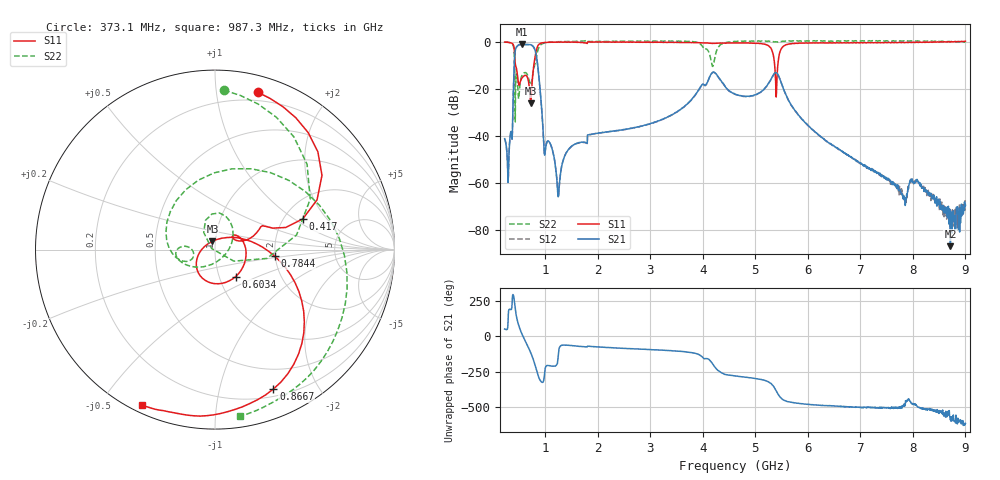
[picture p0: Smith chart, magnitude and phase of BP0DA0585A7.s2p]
!Agilent Technologies,E8358A,US41080443,A.07.50.56
!Agilent E8358A: A.07.50.56
!Date: Friday, November 10, 2017 15:52:36
!Correction: S11(Full 2 Port(1,2))
!S21(Full 2 Port(1,2))
!S12(Full 2 Port(1,2))
!S22(Full 2 Port(1,2))
!S2P File: Measurements: S11, S21, S12, S22:
# Hz S  dB  R 50
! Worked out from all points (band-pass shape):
!   1601 points, 225 MHz to 9 GHz, reference 50 ohm
!   highest |S21| = -1.21 dB at 559.5 MHz (marker M1); lowest = -86.9 dB at 8.715 GHz (marker M2)
!   |S21| within 3 dB of the highest: 425.6 MHz to 812.3 MHz (386.7 MHz wide, 62.5 % of centre)
!   lowest |S11| = -26.2 dB at 724.1 MHz (marker M3), VSWR 1.10, Z = 48.4 + j4.55 ohm
!   |S11| at or under -10 dB: 432.4 MHz to 781.6 MHz (349.3 MHz wide, 57.5 % of centre); 5.368 GHz to 5.428 GHz (59.98 MHz wide, 1.11 % of centre)
!   |S22| runs from -34.1 to 0.5 dB; largest |S21 - S12| = 0.0083
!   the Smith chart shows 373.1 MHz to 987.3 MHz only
!   S11 on the Smith chart (normalised r, x): 373.1 MHz: 0.13, +1.30; 417 MHz: 2.52, +1.18; 603.4 MHz: 1.20, -0.37; 784.4 MHz: 1.98, -0.16; 866.7 MHz: 0.27, -1.47; 987.3 MHz: 0.03, -0.64
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2.25e8  -0.22 138.0  -41.28 52.7  -41.32 52.7  -0.15 148.8
3.237188e8  -0.45 105.1  -41.87 -167.8  -41.98 -167.4  -0.43 119.9
3.730781e8  -0.83 74.8  -38.59 -86.4  -38.67 -86.2  -1.02 86.7
4.169531e8  -5.70 19.3  -6.28 -131.4  -6.36 -131.3  -10.67 -9.7
4.937344e8  -18.39 28.5  -1.42 78.2  -1.50 78.3  -24.34 -56.8
5.595469e8  -15.33 1.7  -1.21 13.9  -1.29 14.0  -14.20 -157.6
6.034219e8  -14.45 -52.5  -1.22 -21.0  -1.30 -21.0  -13.23 -170.1
7.240781e8  -26.21 106.6  -1.37 -115.8  -1.44 -115.7  -18.29 -166.4
7.844062e8  -9.53 -6.2  -2.57 -177.0  -2.63 -177.0  -11.27 169.7
8.666719e8  -1.49 -67.3  -12.43 79.1  -12.48 79.3  -3.16 5.3
9.873281e8  -0.40 -115.1  -48.28 107.0  -48.26 106.5  -0.55 -81.6
1.250578e9  -0.21 -154.1  -65.69 -118.1  -65.60 -122.0  -0.06 -120.7
1.689328e9  -0.37 166.8  -42.75 -70.5  -42.85 -70.4  0.20 -126.7
3.153656e9  -0.28 146.0  -33.70 -95.4  -33.73 -94.8  0.22 -152.8
4.140844e9  -0.71 117.1  -14.44 -171.3  -14.57 -171.0  -6.45 123.4
4.321828e9  -0.62 113.8  -15.88 112.0  -16.04 112.0  -1.64 -88.2
4.6125e9  -0.58 104.2  -22.34 81.6  -22.35 82.0  0.05 -124.3
5.396766e9  -23.57 -78.8  -13.16 -23.4  -13.21 -23.6  -0.11 -142.8
6.076828e9  -0.62 79.9  -37.26 -120.6  -37.32 -121.2  0.19 -152.7
7.541156e9  -0.36 43.9  -58.70 -142.0  -58.56 -143.4  0.23 -164.2
8.714812e9  -0.07 39.0  -86.94 131.1  -74.62 164.4  -0.06 -171.8
9e9  0.12 43.4  -69.57 107.1  -69.94 99.6  -0.19 -178.9
